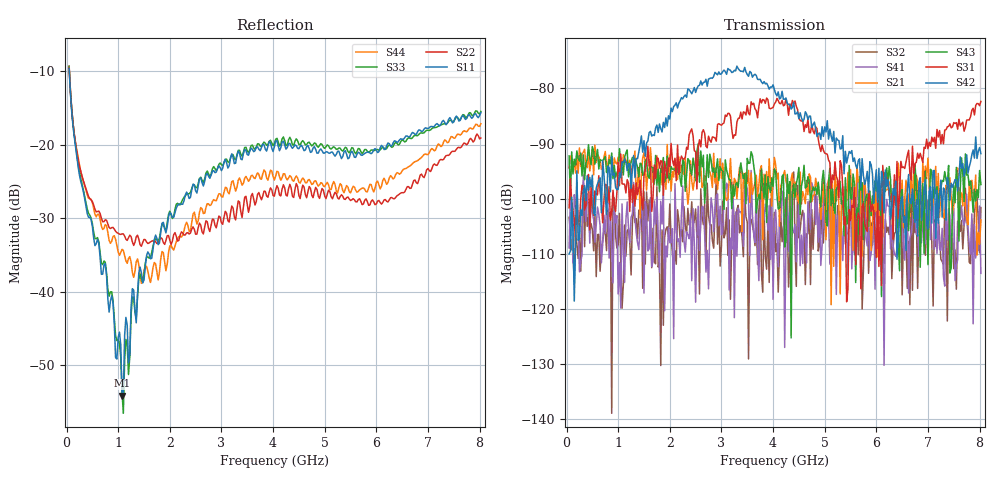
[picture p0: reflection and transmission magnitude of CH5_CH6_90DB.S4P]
!Agilent Technologies,E5071C,MY46316741,A.11.02
!Date: Mon Jun 01 10:12:31 2026
!Data & Calibration Information:
!1:CH5 INPUT 2:CH5 OUTPUT 3:CH6 INPUT 4:CH6 OUTPUT
!Freq	S11:SOLT4(ON)	S12:SOLT4(ON)	S13:SOLT4(ON)	S14:SOLT4(ON)
!	S21:SOLT4(ON)	S22:SOLT4(ON)	S23:SOLT4(ON)	S24:SOLT4(ON)
!	S31:SOLT4(ON)	S32:SOLT4(ON)	S33:SOLT4(ON)	S34:SOLT4(ON)
!	S41:SOLT4(ON)	S42:SOLT4(ON)	S43:SOLT4(ON)	S44:SOLT4(ON)
!PortZ  Port1:50+j0  Port2:50+j0  Port3:50+j0  Port4:50+j0
!Above PortZ is port z conversion or system Z0 setting when saving the data.
!When reading, reference impedance value at option line is always used.
# Hz S dB R 50
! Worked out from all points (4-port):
!   320 points, 50 MHz to 8.025 GHz, reference 50 ohm
!   strongest paths, dB at 50 MHz, 2.05 GHz, 4.05 GHz, 6.05 GHz, 8.025 GHz:
!     S42: -110.0, -84.2, -80.9, -94.5, -91.8
!     S31: -101.6, -92.9, -82.5, -112.3, -82.3
!     S43: -92.3, -94.6, -95.1, -101.9, -97.4
!     S21: -94.4, -95.1, -93.8, -96.2, -103.8
!     S41: -108.9, -105.4, -102.0, -102.2, -113.5
!     S32: -103.4, -109.8, -109.6, -111.3, -101.6
!   lowest |S11| = -54.1 dB at 1.075 GHz (marker M1), VSWR 1.00, Z = 50 + j0.196 ohm
!   |S11| at or under -10 dB: 52.66 MHz to end of sweep
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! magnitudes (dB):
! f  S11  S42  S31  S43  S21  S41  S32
! 50 MHz  -9.6  -110.0  -101.6  -92.3  -94.4  -108.9  -103.4
! 325 MHz  -26.4  -98.7  -97.8  -92.1  -91.6  -95.7  -97.0
! 1.075 GHz  -54.1  -93.3  -97.3  -93.4  -95.3  -101.0  -119.9
! 1.15 GHz  -43.5  -93.3  -99.0  -91.7  -93.4  -103.8  -110.4
! 1.425 GHz  -36.7  -90.2  -96.6  -93.6  -103.5  -104.4  -102.8
! 2.6 GHz  -24.5  -78.6  -90.6  -91.3  -94.2  -104.6  -98.2
! 8.025 GHz  -15.7  -91.8  -82.3  -97.4  -103.8  -113.5  -101.6
